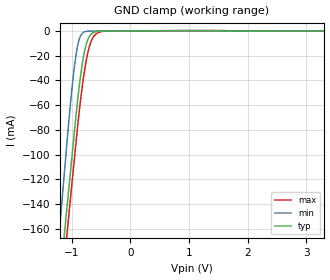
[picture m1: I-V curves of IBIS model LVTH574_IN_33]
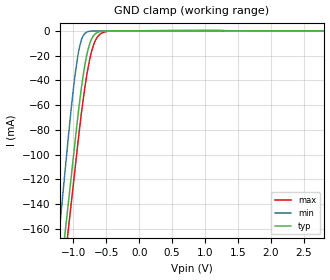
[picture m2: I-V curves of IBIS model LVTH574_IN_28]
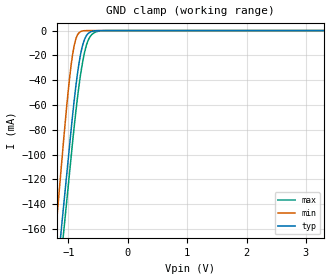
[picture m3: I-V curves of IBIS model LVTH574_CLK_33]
| TEXAS INSTRUMENTS INCORPORATED
| Standard Linear and Logic Group
| IBIS Model of SN74LVTH574
| 3.3-V ABT OCTAL EDGE-TRIGGERED D-TYPE FLIP-FLOPS WITH 3-STATE OUTPUTS
| This file contains package information for the following:
|  SSOP 20-pin (DB) package as [Component] LVTH574_DB
|  SOIC 20-pin (DW) package as [Component] LVTH574_DW
|  TSSOP 20-pin (PW) package as [Component] LVTH574_PW
|  VFBGA 20-pin (GQN) package as [component] LVTH574_GQN
| This device can be powered at the following Vccs:
|  3.3 volt Vcc
|  2.8 volt Vcc
| This file provides unique models under the [Model Selector] for each Vcc.
| For operation at a specific Vcc, select the appropriate model after each
| [Model Selector] keyword.
[IBIS Ver]   3.2
[Comment char]  |_char
[File Name]   sn74lvth574.ibs
[File Rev]   1.1 | x_die
[Date]   June 26, 2002
[Source]   Data created from TI-SPICE simulations at TI-SLL.
[Notes]   The following is an IBIS list for the LVTH574.
   Please contact sllibis@ti.com with questions and
   comments concerning SLL IBIS models.
   Non-monotonic data in input due to bus-hold.
   As there is no power clamp diode in the Input and Output
   Models, we removed the Pwr Clamp table data from those
   Models.
   Due to the fact that the Device is 5-V Input/Output
   tolarent, the output model has some Non-Monotonic Warnings.
[Disclaimer] Property of Texas Instruments Incorporated.  Unauthorized
   reproduction and/or distribution is strictly prohibited.
   This product is protected under copyright law.
   Created  2002, (C) Copyright  2002, Texas Instruments
   Incorporated, All Rights Reserved
   UNLESS THERE IS A SIGNED, WRITTEN AGREEMENT TO THE
   CONTRARY, TEXAS INSTRUMENTS (TI) IS PROVIDING THE IBIS
   MODELS  AND WITHOUT ANY WARRANTY, EXPRESSED OR
   IMPLIED.  TI assumes no liability for:
   1) the accuracy of the IBIS models provided to your
   company;
   2) the proper functioning of these IBIS Models in your
   design or for any resulting applications; or
   3) infringement of patents, copyrights or intellectual
   property rights resulting from your use of these IBIS
   models.
   TI provides IBIS Models as a service to our customers.
   You and your company shall not distribute, sell or give
   these models to anyone else without prior written
   permission from TI.
   TI reserves the right to make changes to our products or
   to discontinue any semiconductor product or service
   without notice, and advises our customers to obtain the
   latest version of relevant information to verify, before
   placing orders, that the information being relied on is
   current.
   Please be aware that your receipt and use of the IBIS
   information provided shall serve as acceptance of these
   terms and conditions.  If you do not accept these terms,
   you should return or destroy the IBIS models and any
   other accompanying information immediately.
| Component LVTH574_DB 20-pin SSOP
[Component]   LVTH574_DB
[Manufacturer]   Texas Instruments, Inc.
[Package]
|   typ   min   max
R_pkg   4.000e-02   3.500e-02   5.100e-02
L_pkg   3.495e-09   3.035e-09   4.314e-09
C_pkg   4.200e-13   3.460e-13   5.020e-13
[Pin]   signal_name   model_name   R_pin   L_pin   C_pin
1   NOE   LVTH574_OE   4.900e-02   4.310e-09   5.020e-13
2   1D   LVTH574_IN   4.800e-02   3.903e-09   4.870e-13
3   2D   LVTH574_IN   3.500e-02   3.189e-09   3.960e-13
4   3D   LVTH574_IN   3.500e-02   3.036e-09   3.470e-13
5   4D   LVTH574_IN   3.500e-02   3.035e-09   3.670e-13
6   5D   LVTH574_IN   3.500e-02   3.035e-09   3.670e-13
7   6D   LVTH574_IN   3.500e-02   3.036e-09   3.470e-13
8   7D   LVTH574_IN   3.500e-02   3.189e-09   3.970e-13
9   8D   LVTH574_IN   4.700e-02   3.899e-09   4.880e-13
10   GND   GND   5.100e-02   4.314e-09   5.000e-13
11   CLK   LVTH574_CLK   5.100e-02   4.314e-09   5.000e-13
12   8Q   LVTH574_OUT   4.700e-02   3.899e-09   4.880e-13
13   7Q   LVTH574_OUT   3.500e-02   3.189e-09   3.970e-13
14   6Q   LVTH574_OUT   3.500e-02   3.036e-09   3.460e-13
15   5Q   LVTH574_OUT   3.500e-02   3.035e-09   3.670e-13
16   4Q   LVTH574_OUT   3.500e-02   3.035e-09   3.670e-13
17   3Q   LVTH574_OUT   3.500e-02   3.036e-09   3.460e-13
18   2Q   LVTH574_OUT   3.500e-02   3.189e-09   3.970e-13
19   1Q   LVTH574_OUT   4.700e-02   3.899e-09   4.880e-13
20   VCC   POWER   5.100e-02   4.314e-09   5.020e-13
| Component LVTH574_DW 20-pin SOIC
[Component]   LVTH574_DW
[Manufacturer]   Texas Instruments, Inc.
[Package]
|   typ   min   max
R_pkg   3.800e-02   3.300e-02   4.500e-02
L_pkg   5.012e-09   4.110e-09   6.349e-09
C_pkg   7.170e-13   5.300e-13   8.680e-13
[Pin]   signal_name   model_name   R_pin   L_pin   C_pin
1   NOE   LVTH574_OE   4.200e-02   6.336e-09   8.650e-13
2   1D   LVTH574_IN   4.300e-02   5.542e-09   8.670e-13
3   2D   LVTH574_IN   3.400e-02   4.714e-09   7.320e-13
4   3D   LVTH574_IN   3.400e-02   4.377e-09   5.910e-13
5   4D   LVTH574_IN   3.600e-02   4.130e-09   5.330e-13
6   5D   LVTH574_IN   3.500e-02   4.111e-09   5.300e-13
7   6D   LVTH574_IN   3.400e-02   4.284e-09   5.830e-13
8   7D   LVTH574_IN   3.400e-02   4.634e-09   7.260e-13
9   8D   LVTH574_IN   4.000e-02   5.518e-09   8.650e-13
10   GND   GND   4.300e-02   6.349e-09   8.660e-13
11   CLK   LVTH574_CLK   4.100e-02   6.281e-09   8.610e-13
12   8Q   LVTH574_OUT   4.500e-02   5.561e-09   8.680e-13
13   7Q   LVTH574_OUT   3.300e-02   4.778e-09   7.420e-13
14   6Q   LVTH574_OUT   3.500e-02   4.414e-09   5.960e-13
15   5Q   LVTH574_OUT   3.500e-02   4.110e-09   5.330e-13
16   4Q   LVTH574_OUT   3.600e-02   4.130e-09   5.330e-13
17   3Q   LVTH574_OUT   3.400e-02   4.377e-09   5.910e-13
18   2Q   LVTH574_OUT   3.400e-02   4.714e-09   7.310e-13
19   1Q   LVTH574_OUT   4.300e-02   5.569e-09   8.680e-13
20   VCC   POWER   4.200e-02   6.308e-09   8.640e-13
| Component LVTH574_PW 20-pin TSSOP
[Component]   LVTH574_PW
[Manufacturer]   Texas Instruments, Inc.
[Package]
|   typ   min   max
R_pkg   5.000e-02   4.200e-02   6.000e-02
L_pkg   2.802e-09   2.248e-09   3.553e-09
C_pkg   3.170e-13   2.020e-13   4.430e-13
[Pin]   signal_name   model_name   R_pin   L_pin   C_pin
1   NOE   LVTH574_OE   5.500e-02   3.461e-09   4.400e-13
2   1D   LVTH574_IN   5.500e-02   3.150e-09   4.010e-13
3   2D   LVTH574_IN   4.200e-02   2.619e-09   3.020e-13
4   3D   LVTH574_IN   4.500e-02   2.273e-09   2.020e-13
5   4D   LVTH574_IN   4.500e-02   2.248e-09   2.240e-13
6   5D   LVTH574_IN   4.500e-02   2.273e-09   2.260e-13
7   6D   LVTH574_IN   4.400e-02   2.323e-09   2.050e-13
8   7D   LVTH574_IN   4.600e-02   2.704e-09   3.070e-13
9   8D   LVTH574_IN   6.000e-02   3.265e-09   4.110e-13
10   GND   GND   5.700e-02   3.506e-09   4.360e-13
11   CLK   LVTH574_CLK   5.800e-02   3.553e-09   4.370e-13
12   8Q   LVTH574_OUT   5.800e-02   3.193e-09   4.050e-13
13   7Q   LVTH574_OUT   4.200e-02   2.704e-09   3.110e-13
14   6Q   LVTH574_OUT   4.600e-02   2.392e-09   2.100e-13
15   5Q   LVTH574_OUT   4.700e-02   2.334e-09   2.290e-13
16   4Q   LVTH574_OUT   4.700e-02   2.300e-09   2.270e-13
17   3Q   LVTH574_OUT   4.700e-02   2.349e-09   2.070e-13
18   2Q   LVTH574_OUT   4.500e-02   2.677e-09   3.060e-13
19   1Q   LVTH574_OUT   6.000e-02   3.235e-09   4.060e-13
20   VCC   POWER   5.600e-02   3.487e-09   4.430e-13
| Component LVTH574_GQN 20-pin VFBGA
[Component]   LVTH574_GQN
[Manufacturer] Texas Instruments, Inc.
[Package]
|   typ   min   max
R_pkg   4.300e-02   3.300e-02   6.100e-02
L_pkg   1.317e-09   8.960e-10   2.088e-09
C_pkg   1.130e-13   6.400e-14   1.900e-13
[Pin]   signal_name   model_name   R_pin   L_pin   C_pin
A2   1NOE   LVTH574_OE   3.800e-02   1.199e-09   1.210e-13
A1   1D   LVTH574_IN   4.000e-02   1.067e-09   1.020e-13
B3   2D   LVTH574_IN   6.100e-02   1.999e-09   1.900e-13
B1   3D   LVTH574_IN   3.300e-02   9.630e-10   7.100e-14
C2   4D   LVTH574_IN   4.900e-02   1.523e-09   1.230e-13
C1   5D   LVTH574_IN   3.300e-02   8.960e-10   6.400e-14
D3   6D   LVTH574_IN   6.100e-02   1.899e-09   1.640e-13
D1   7D   LVTH574_IN   3.300e-02   8.980e-10   6.700e-14
E2   8D   LVTH574_IN   4.900e-02   1.514e-09   1.280e-13
E1   GND   GND   3.600e-02   1.006e-09   9.400e-14
E3   CLK   LVTH574_CLK   4.900e-02   1.683e-09   1.460e-13
E4   8Q   LVTH574_OUT   3.300e-02   1.121e-09   8.900e-14
D2   7Q   LVTH574_OUT   6.100e-02   2.088e-09   1.730e-13
D4   6Q   LVTH574_OUT   3.300e-02   1.027e-09   7.100e-14
C3   5Q   LVTH574_OUT   4.900e-02   1.558e-09   1.240e-13
C4   4Q   LVTH574_OUT   3.300e-02   9.280e-10   6.700e-14
B2   3Q   LVTH574_OUT   6.100e-02   1.921e-09   1.770e-13
B4   2Q   LVTH574_OUT   3.300e-02   9.010e-10   7.700e-14
A4   1Q   LVTH574_OUT   3.700e-02   9.900e-10   9.800e-14
A3   VCC   POWER   3.500e-02   1.168e-09   1.190e-13
| Model LVTH574_IN
[Model Selector]   LVTH574_IN
LVTH574_IN_33   3.3 volt Vcc
LVTH574_IN_28   2.8 volt Vcc
| Model LVTH574_CLK
[Model Selector]   LVTH574_CLK
LVTH574_CLK_33   3.3 volt Vcc
LVTH574_CLK_28   2.8 volt Vcc
| Model LVTH574_OE
[Model Selector]   LVTH574_OE
LVTH574_OE_33   3.3 volt Vcc
LVTH574_OE_28   2.8 volt Vcc
| Model LVTH574_OUT
[Model Selector]   LVTH574_OUT
LVTH574_OUT_33   3.3 volt Vcc
LVTH574_OUT_28   2.8 volt Vcc
| Models and submodels in the file (8): LVTH574_IN_33 (Input), LVTH574_IN_28 (Input), LVTH574_CLK_33 (Input), LVTH574_CLK_28 (Input), LVTH574_OE_33 (Input), LVTH574_OE_28 (Input), LVTH574_OUT_33 (3-state), LVTH574_OUT_28 (3-state)
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[Model]   LVTH574_IN_33
Model_type  Input
Vinl = 0.8
Vinh = 2.34
| variable   typ   min   max
C_comp   3.80pF   3.14pF   5.36pF
[Temperature Range]   40   -40   100
| Ambient temperature   25   -40   85
[Voltage range]   3.3   3   3.6
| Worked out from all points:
|   GND clamp passes 1 mA (typ) near -0.62 V on its own axis
[GND Clamp]
| LVTH574_IN_33
|   Voltage   I(typ)   I(min)   I(max)
-5.5V     -2.408A    -2.65A     -2.407A
-1.22V    -209.4mA   -166.2mA   -230.2mA
-1.19V    -194.8mA   -149.4mA   -215.7mA
-1.125V   -163.2mA   -113.2mA   -184.4mA
-1.075V   -138.9mA   -85.44mA   -160.3mA
-975mV    -90.33mA   -36.32mA   -112.1mA
-900mV    -55.43mA   -11.64mA   -76.61mA
-825mV    -27.57mA   -2.159mA   -45.81mA
-775mV    -14.79mA   -632.4uA   -29.53mA
-650mV    -1.834mA   -141.2uA   -6.249mA
-405mV    -96.3uA    -83.9uA    -154.2uA
3.3V      19.45pA    12.56pA    -1.096uA
[Model]   LVTH574_IN_28
Model_type  Input
Vinl = 0.8
Vinh = 2.0
| variable   typ   min   max
C_comp   3.87pF   3.20pF   5.30pF
[Temperature Range]   40   -40   100
| Ambient temperature   25   -40   85
[Voltage range]   2.8   2.7   2.9
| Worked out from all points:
|   GND clamp passes 1 mA (typ) near -0.62 V on its own axis
[GND Clamp]
| LVTH574_IN_28
|   Voltage   I(typ)   I(min)   I(max)
-5.5V     -2.408A    -2.65A     -2.407A
-1.22V    -209.4mA   -166.2mA   -230.2mA
-1.205V   -202.1mA   -157.8mA   -222.9mA
-1.125V   -163.2mA   -113.2mA   -184.4mA
-1.075V   -138.9mA   -85.42mA   -160.3mA
-975mV    -90.32mA   -36.3mA    -112.1mA
-900mV    -55.42mA   -11.62mA   -76.6mA
-800mV    -20.4mA    -1.145mA   -37.03mA
-675mV    -2.832mA   -140.1uA   -8.833mA
-575mV    -458.4uA   -111.8uA   -2.088mA
-425mV    -91.65uA   -80.29uA   -190.6uA
2.8V      16.5pA     10.34pA    -1.623nA
[Model]   LVTH574_CLK_33
Model_type  Input
Vinl = 0.8
Vinh = 2.34
| variable   typ   min   max
C_comp   4.04pF   3.22pF   5.46pF
[Temperature Range]   40   -40   100
| Ambient temperature   25   -40   85
[Voltage range]   3.3   3   3.6
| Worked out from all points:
|   GND clamp passes 1 mA (typ) near -0.62 V on its own axis
[GND Clamp]
| LVTH574_CLK_33
|   Voltage   I(typ)   I(min)   I(max)
-5.5V     -2.407A    -2.649A    -2.406A
-1.22V    -209.3mA   -166mA     -230mA
-1.205V   -202mA     -157.6mA   -222.8mA
-1.125V   -163.1mA   -113mA     -184.2mA
-1.075V   -138.8mA   -85.25mA   -160.1mA
-975mV    -90.17mA   -36.12mA   -112mA
-900mV    -55.28mA   -11.44mA   -76.47mA
-825mV    -27.42mA   -1.98mA    -45.67mA
-775mV    -14.64mA   -464.8uA   -29.41mA
-650mV    -1.684mA   -2.076uA   -6.132mA
-395mV    -1.224uA   -43.32pA   -35.77uA
3.3V      16.15pA    8.657pA    1.272nA
